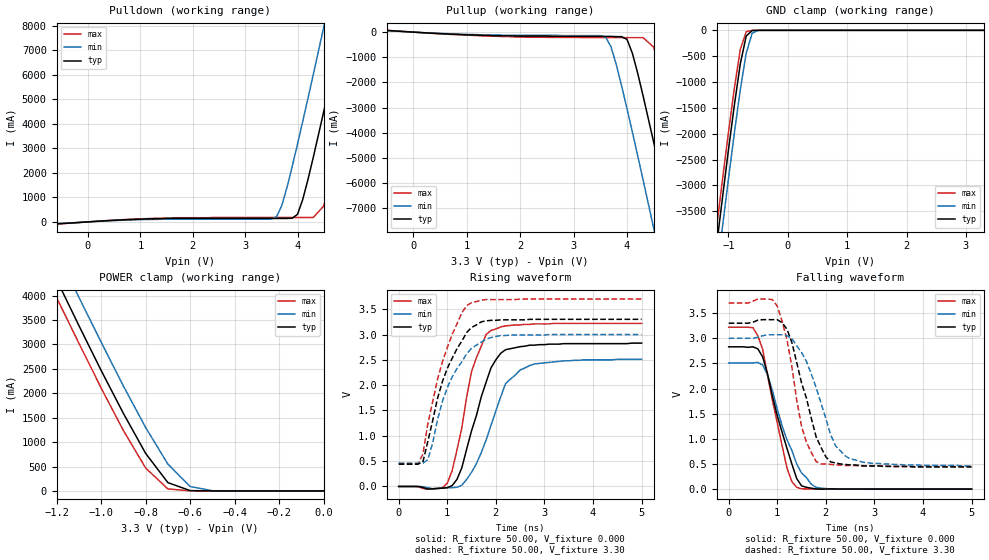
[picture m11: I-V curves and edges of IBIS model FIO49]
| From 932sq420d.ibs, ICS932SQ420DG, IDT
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|   Model FIO49
[Model]   FIO49
Model_type   I/O
Polarity   Non-Inverting
Enable   Active-High
Vinl =   0.80V
Vinh =   2.00V
Vmeas =   1.50V
C_comp   3.40pF   2.85pF   3.95pF
[Temperature Range]   27.00   70.00   0.000
[Voltage Range]   3.30V   3.00V   3.70V
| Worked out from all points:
|   slope of the pulldown table from 0 to 0.495 V, typ, clamps not added: 7.81 ohm
|   slope of the pullup table from 0 to 0.495 V, typ, clamps not added: 8.42 ohm
|   GND clamp passes 1 mA (typ) near -0.52 V on its own axis
|   POWER clamp passes 1 mA (typ) near -0.51 V on its own axis
|   rising waveform, R_fixture 50.00, V_fixture 0.000: 20-80 % time 520ps typ, 568ps min, 434ps max; typ from 0 V to 2.83 V
|   rising waveform, R_fixture 50.00, V_fixture 3.30: 20-80 % time 576ps typ, 597ps min, 547ps max; typ from 0.44 V to 3.3 V
|   falling waveform, R_fixture 50.00, V_fixture 0.000: 20-80 % time 473ps typ, 515ps min, 410ps max; typ from 2.83 V to 0 V
|   falling waveform, R_fixture 50.00, V_fixture 3.30: 20-80 % time 465ps typ, 532ps min, 368ps max; typ from 3.3 V to 0.44 V
[Pulldown]
| voltage   I(typ)   I(min)   I(max)
|  -3.30   0.000A   -0.40A   0.000A
|  -3.10   0.000A   0.000A   0.000A
|  -2.90   0.000A   0.000A   0.000A
|  -2.70   0.000A   -10.00mA   0.000A
|  -2.50   0.000A   0.000A   0.000A
|  -2.30   0.000A   0.000A   0.000A
|  -2.10   0.000A   0.000A   0.000A
|  -1.90   0.000A   0.000A   0.000A
|  -1.70   -3.00mA   -2.00mA   -3.00mA
|  -1.50   -4.00mA   -4.00mA   -3.00mA
|  -1.00   -10.00mA   -8.00mA   -13.00mA
|  -0.90   -15.00mA   -11.00mA   -20.00mA
|  -0.80   -28.50mA   -17.00mA   -43.80mA
|  -0.70   -66.30mA   -32.60mA   -91.83mA
-600mV    -80.27mA   -61.2mA    -87.64mA
1.3V      130mA      100mA      150mA
3.6V      140mA      210mA      180mA
3.7V      140mA      670mA      180mA
4V        310mA      3.18A      180mA
4.1V      920mA      4.11A      180mA
4.3V      2.63A      6.01A      180mA
4.5V      4.5A       7.94A      650mA
4.7V      6.42A      9.88A      2.3A
4.9V      8.36A      11.84A     4.17A
5.3V      12.28A     15.78A     8.04A
6.6V      25.18A     28.67A     20.9A
[Pullup]
| voltage   I(typ)   I(min)   I(max)
|  -3.30   0.000A   0.000A   10.00mA
|  -3.10   10.00mA   10.00mA   0.000A
|  -2.90   0.000A   0.000A   10.00mA
|  -2.70   0.000A   0.000A   0.000A
|  -2.50   0.000A   0.000A   10.00mA
|  -2.30   0.000A   10.00mA   10.00mA
|  -2.10   0.000A   10.00mA   0.000A
|  -1.90   0.000A   0.000A   0.000A
|  -1.70   3.00mA   3.00mA   4.00mA
|  -1.50   4.00mA   4.00mA   4.00mA
|  -1.00   10.00mA   7.00mA   15.00mA
|  -0.90   15.00mA   10.00mA   19.00mA
|  -0.80   25.60mA   16.00mA   39.70mA
|  -0.70   58.40mA   28.40mA   89.84mA
|  -0.60   79.27mA   56.12mA   88.51mA
-500mV    67.38mA    59.46mA    73.94mA
3.6V      -170mA     -200mA     -220mA
3.7V      -170mA     -580mA     -220mA
4V        -290mA     -3.05A     -220mA
4.1V      -840mA     -3.97A     -220mA
4.3V      -2.53A     -5.87A     -220mA
4.5V      -4.39A     -7.81A     -600mA
4.7V      -6.32A     -9.76A     -2.23A
4.9V      -8.26A     -11.72A    -4.09A
5.1V      -10.23A    -13.7A     -6.02A
5.3V      -12.2A     -15.68A    -7.97A
6.6V      -25.15A    -28.64A    -20.87A
[GND_clamp]
| voltage   I(typ)   I(min)   I(max)
-3.3V     -24.71A    -25.24A    -24.39A
-1.2V     -4.17A     -4.73A     -3.82A
-1.1V     -3.24A     -3.8A      -2.89A
-1V       -2.32A     -2.88A     -1.98A
-900mV    -1.45A     -1.99A     -1.12A
-800mV    -650mA     -1.15A     -370mA
-700mV    -110mA     -440mA     -25.27mA
-600mV    -4.15mA    -55.1mA    -810uA
-500mV    -170uA     -2.39mA    -69.26uA
3.3V      35.68uA    29.04uA    51.26uA
[POWER_clamp]
| voltage   I(typ)   I(min)   I(max)
-3.3V     24.87A     25.42A     24.53A
-1.2V     4.33A      4.91A      3.96A
-1.1V     3.39A      3.97A      3.03A
-1V       2.47A      3.05A      2.11A
-900mV    1.59A      2.15A      1.24A
-800mV    770mA      1.3A       470mA
-700mV    170mA      550mA      41.26mA
-600mV    6.65mA     90.58mA    760uA
-500mV    180uA      4.16mA     62.13uA
0V        35.68nA    24.08nA    51.3nA
[Ramp]
| variable   typ   min   max
dV/dt_r   1.70/0.50n   1.51/0.61n   1.93/0.43n
dV/dt_f   1.72/0.45n   1.52/0.55n   1.95/0.37n
R_load = 50.00
[Rising Waveform]
R_fixture = 50.00
V_fixture = 0.000
V_fixture_min = 0.000
V_fixture_max = 0.000
| time   V(typ)   V(min)   V(max)
0s        0V         0V         0V
600ps     -51.33mV   -24.59mV   -53.5mV
1ns       -22.94mV   -28.24mV   63.39mV
1.2ns     140mV      -16.85mV   720mV
1.5ns     1.1V       280mV      2.27V
1.8ns     2.06V      920mV      3V
1.9ns     2.34V      1.21V      3.08V
2.2ns     2.7V       2.03V      3.17V
2.7ns     2.79V      2.39V      3.2V
5ns       2.83V      2.51V      3.22V
[Rising Waveform]
R_fixture = 50.00
V_fixture = 3.30
V_fixture_min = 3.00
V_fixture_max = 3.70
| time   V(typ)   V(min)   V(max)
0s        440mV      460mV      450mV
400ps     440mV      460mV      450mV
500ps     490mV      460mV      640mV
600ps     890mV      530mV      1.24V
900ps     2.07V      1.68V      2.46V
1.1ns     2.53V      2.16V      3V
1.4ns     3.04V      2.62V      3.57V
1.7ns     3.25V      2.85V      3.68V
2.1ns     3.29V      2.98V      3.69V
5ns       3.3V       3V         3.7V
[Falling Waveform]
R_fixture = 50.00
V_fixture = 0.000
V_fixture_min = 0.000
V_fixture_max = 0.000
| time   V(typ)   V(min)   V(max)
0s        2.83V      2.51V      3.22V
500ps     2.83V      2.51V      3.21V
600ps     2.79V      2.52V      3.05V
700ps     2.63V      2.47V      2.78V
800ps     2.29V      2.27V      2.26V
1.2ns     810mV      980mV      420mV
1.4ns     210mV      500mV      35.5mV
1.7ns     18.07mV    95.13mV    3.66mV
1.9ns     -1.67mV    18.88mV    2.39mV
5ns       62.32uV    100uV      25.13uV
[Falling Waveform]
R_fixture = 50.00
V_fixture = 3.30
V_fixture_min = 3.00
V_fixture_max = 3.70
| time   V(typ)   V(min)   V(max)
0s        3.3V       3V         3.7V
800ps     3.37V      3.07V      3.78V
1ns       3.37V      3.07V      3.64V
1.2ns     3.18V      3.05V      2.97V
1.5ns     2.11V      2.72V      1.25V
1.8ns     1.04V      2.02V      550mV
2ns       640mV      1.4V       500mV
2.2ns     520mV      860mV      480mV
2.5ns     480mV      600mV      470mV
5ns       440mV      460mV      450mV
